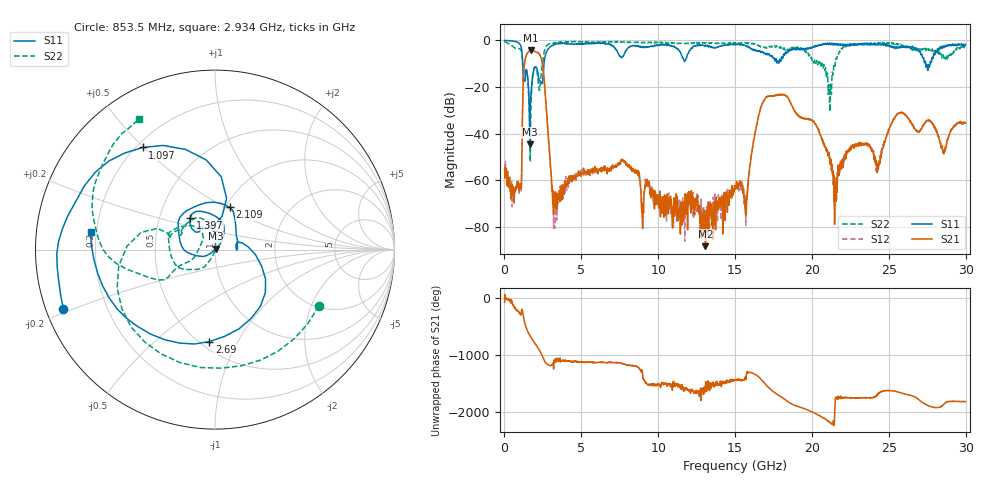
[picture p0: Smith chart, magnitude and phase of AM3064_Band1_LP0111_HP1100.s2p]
# Hz S DB R 50.0
!freq dBS11 angS11 dBS21 angS21 dBS12 angS12 dBS22 angS22
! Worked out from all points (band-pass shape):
!   1600 points, 10 MHz to 29.98 GHz, reference 50 ohm
!   highest |S21| = -4.32 dB at 1.716 GHz (marker M1); lowest = -88.2 dB at 13.07 GHz (marker M2)
!   |S21| within 3 dB of the highest: 1.376 GHz to 2.376 GHz (1 GHz wide, 53.3 % of centre)
!   lowest |S11| = -44.6 dB at 1.641 GHz (marker M3), VSWR 1.01, Z = 50.3 + j0.496 ohm
!   |S11| at or under -10 dB: 1.187 GHz to 2.574 GHz (1.388 GHz wide, 73.8 % of centre); 27.4 GHz to 27.68 GHz (282.6 MHz wide, 1.03 % of centre)
!   |S22| runs from -52.0 to -0.3 dB; largest |S21 - S12| = 0.011
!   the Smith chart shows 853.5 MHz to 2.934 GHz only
!   S11 on the Smith chart (normalised r, x): 853.5 MHz: 0.05, -0.19; 1.097 GHz: 0.22, +0.50; 1.397 GHz: 0.71, +0.27; 2.109 GHz: 1.04, +0.52; 2.69 GHz: 0.56, -0.77; 2.934 GHz: 0.18, +0.07
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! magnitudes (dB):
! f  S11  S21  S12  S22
! 10 MHz  -0.1  -55.1  -57.5  -0.3
! 853.5 MHz  -0.8  -62.4  -63.2  -3.6
! 1.097 GHz  -3.1  -63.5  -64.5  -4.6
! 1.397 GHz  -12.9  -6.9  -6.9  -13.3
! 1.641 GHz  -44.6  -4.5  -4.5  -35.4
! 1.716 GHz  -23.4  -4.3  -4.3  -30.5
! 2.109 GHz  -12.1  -5.1  -5.1  -13.0
! 2.69 GHz  -5.8  -26.3  -26.3  -2.8
! 2.934 GHz  -3.1  -48.1  -48.9  -1.5
! 3.29 GHz  -1.8  -66.9  -68.0  -0.9
! 5.015 GHz  -1.5  -57.2  -57.2  -0.7
! 7.751 GHz  -6.4  -51.6  -51.2  -0.7
! 10 GHz  -2.1  -70.7  -70.1  -0.9
! 13.07 GHz  -2.0  -88.2  -75.5  -1.1
! 15 GHz  -1.9  -62.6  -62.3  -1.4
! 15.72 GHz  -2.4  -73.6  -71.7  -1.3
! 17.03 GHz  -5.9  -24.2  -24.4  -3.4
! 19.99 GHz  -3.3  -34.4  -34.3  -8.1
! 21.15 GHz  -1.4  -51.0  -51.4  -28.1
! 21.53 GHz  -1.6  -63.4  -62.8  -9.1
! 25 GHz  -2.0  -38.5  -38.1  -1.2
! 29.98 GHz  -1.7  -35.5  -35.4  -3.0
